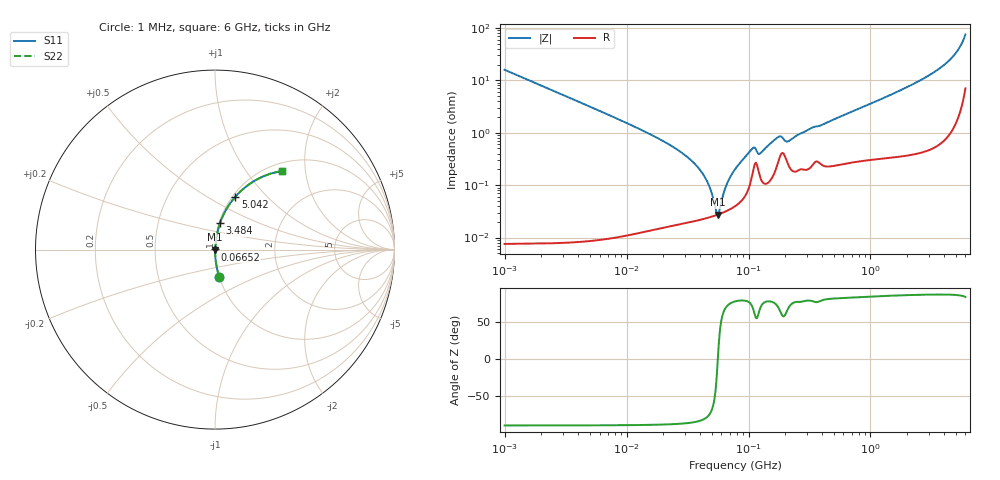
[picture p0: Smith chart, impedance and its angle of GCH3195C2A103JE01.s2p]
!Murata Part Number: GCH3195C2A103JE01
!These Parameters are Measured in Series Mode Connection
!Data Generated on Jun 19, 2026
!  o--ll--o
!Port1  Port2
!  o------o
!Operation Temp=25[degC], DC Bias Voltage=0[V]
!Freq. Start=1000[kHz] Stop=6[GHz] 401[Steps]
# Hz S RI R 50
!Freq.(Hz) S11(Real) S11(Imag) S21(Real) S21(Imag) S12(Real) S12(Imag) S22(Real) S22(Imag)
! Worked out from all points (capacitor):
!   401 points, 1 MHz to 6 GHz, reference 50 ohm
!   read as one part in series: C = 10 nF near 1.044 MHz
!   lowest |Z| = 27.4 mohm at 55.9 MHz (marker M1)
!   series resonance near 55.98 MHz, so ESL is about 810 pH
!   S11 on the Smith chart (normalised r, x): 1 MHz: 1.00, -0.32; 66.52 MHz: 1.00, +0.00; 3.484 GHz: 1.01, +0.31; 5.042 GHz: 1.03, +0.68; 6 GHz: 1.14, +1.49
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1000000  0.0246 -0.1547  0.9754 0.1547  0.9754 0.1547  0.0246 -0.1547
4293785  0.00143 -0.0367  0.9986 0.0367  0.9986 0.0367  0.00143 -0.0367
1.843659e7  0.000206 -0.00764  0.9998 0.00764  0.9998 0.00764  0.000206 -0.00764
2.848316e7  0.000199 -0.00411  0.9998 0.00411  0.9998 0.00411  0.000199 -0.00411
3.8621e7  0.000217 -0.00215  0.9998 0.00215  0.9998 0.00215  0.000217 -0.00215
4.596069e7  0.000238 -0.00113  0.9998 0.00113  0.9998 0.00113  0.000238 -0.00113
4.905945e7  0.000248 -0.000755  0.9998 0.000755  0.9998 0.000755  0.000248 -0.000755
5.351853e7  0.000264 -0.000258  0.9997 0.000258  0.9997 0.000258  0.000264 -0.000258
5.589783e7  0.000273 -8.7e-06  0.9997 8.7e-06  0.9997 8.7e-06  0.000273 -8.7e-06
5.838291e7  0.000284 0.000241  0.9997 -0.000241  0.9997 -0.000241  0.000284 0.000241
6.652088e7  0.000324 0.00101  0.9997 -0.00101  0.9997 -0.00101  0.000324 0.00101
7.745967e7  0.000399 0.00196  0.9996 -0.00196  0.9996 -0.00196  0.000399 0.00196
1.073387e8  0.00159 0.00471  0.9984 -0.00471  0.9984 -0.00471  0.00159 0.00471
1.249896e8  0.0014 0.00378  0.9986 -0.00378  0.9986 -0.00378  0.0014 0.00378
1.732027e8  0.00259 0.00771  0.9974 -0.00771  0.9974 -0.00771  0.00259 0.00771
1.848803e8  0.00395 0.00744  0.9961 -0.00744  0.9961 -0.00744  0.00395 0.00744
2.106508e8  0.00253 0.00632  0.9975 -0.00632  0.9975 -0.00632  0.00253 0.00632
3.325952e8  0.0025 0.0122  0.9975 -0.0122  0.9975 -0.0122  0.0025 0.0122
1.428092e9  0.00591 0.0509  0.9941 -0.0509  0.9941 -0.0509  0.00591 0.0509
3.483508e9  0.0281 0.1485  0.9719 -0.1485  0.9719 -0.1485  0.0281 0.1485
5.04183e9  0.1134 0.2949  0.8866 -0.2949  0.8866 -0.2949  0.1134 0.2949
6e9  0.3709 0.4384  0.6291 -0.4384  0.6291 -0.4384  0.3709 0.4384
